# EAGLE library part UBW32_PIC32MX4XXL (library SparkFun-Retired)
Generic PIC32MX4XXL SparkFun Products None
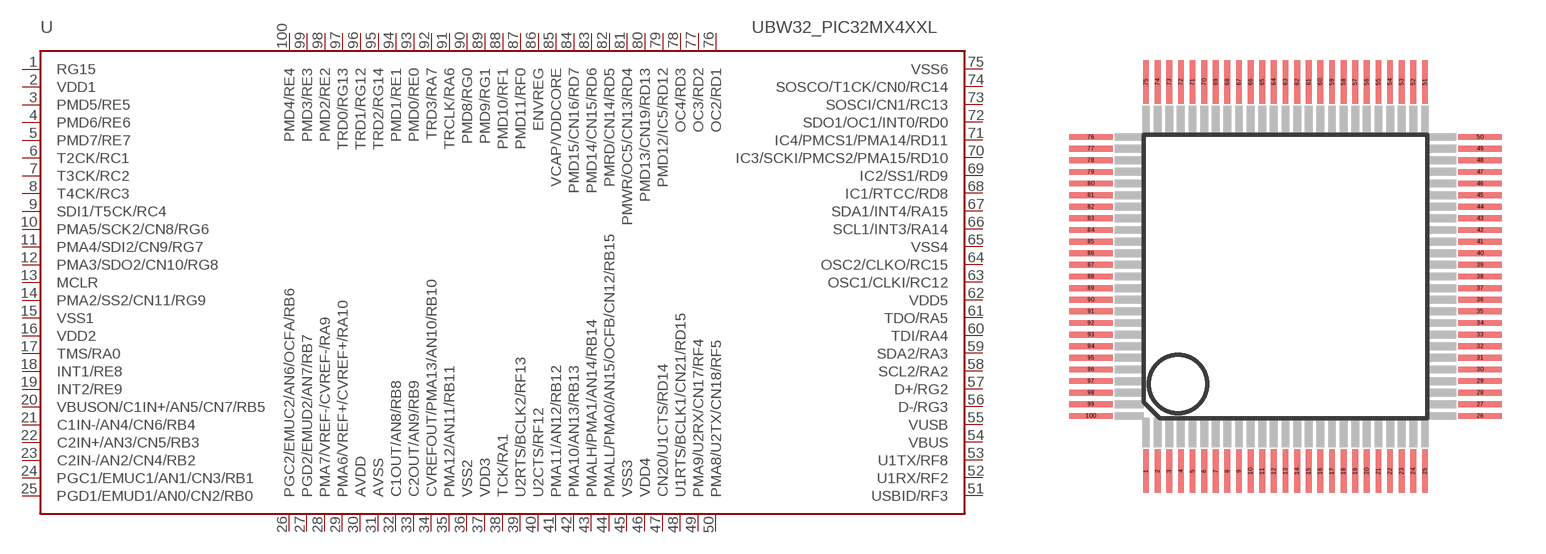
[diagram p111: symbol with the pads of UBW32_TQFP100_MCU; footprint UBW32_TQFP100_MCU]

Designator prefix -

## UBW32_PIC32MX4XXLTQFP100  [UBW32_TQFP100_MCU]
1  RG15
2  VDD1
3  PMD5/RE5
4  PMD6/RE6
5  PMD7/RE7
6  T2CK/RC1
7  T3CK/RC2
8  T4CK/RC3
9  SDI1/T5CK/RC4
10  PMA5/SCK2/CN8/RG6
11  PMA4/SDI2/CN9/RG7
12  PMA3/SDO2/CN10/RG8
13  MCLR
14  PMA2/SS2/CN11/RG9
15  VSS1
16  VDD2
17  TMS/RA0
18  INT1/RE8
19  INT2/RE9
20  VBUSON/C1IN+/AN5/CN7/RB5
21  C1IN-/AN4/CN6/RB4
22  C2IN+/AN3/CN5/RB3
23  C2IN-/AN2/CN4/RB2
24  PGC1/EMUC1/AN1/CN3/RB1
25  PGD1/EMUD1/AN0/CN2/RB0
26  PGC2/EMUC2/AN6/OCFA/RB6
27  PGD2/EMUD2/AN7/RB7
28  PMA7/VREF-/CVREF-/RA9
29  PMA6/VREF+/CVREF+/RA10
30  AVDD
31  AVSS
32  C1OUT/AN8/RB8
33  C2OUT/AN9/RB9
34  CVREFOUT/PMA13/AN10/RB10
35  PMA12/AN11/RB11
36  VSS2
37  VDD3
38  TCK/RA1
39  U2RTS/BCLK2/RF13
40  U2CTS/RF12
41  PMA11/AN12/RB12
42  PMA10/AN13/RB13
43  PMALH/PMA1/AN14/RB14
44  PMALL/PMA0/AN15/OCFB/CN12/RB15
45  VSS3
46  VDD4
47  CN20/U1CTS/RD14
48  U1RTS/BCLK1/CN21/RD15
49  PMA9/U2RX/CN17/RF4
50  PMA8/U2TX/CN18/RF5
51  USBID/RF3
52  U1RX/RF2
53  U1TX/RF8
54  VBUS
55  VUSB
56  D-/RG3
57  D+/RG2
58  SCL2/RA2
59  SDA2/RA3
60  TDI/RA4
61  TDO/RA5
62  VDD5
63  OSC1/CLKI/RC12
64  OSC2/CLKO/RC15
65  VSS4
66  SCL1/INT3/RA14
67  SDA1/INT4/RA15
68  IC1/RTCC/RD8
69  IC2/SS1/RD9
70  IC3/SCKI/PMCS2/PMA15/RD10
71  IC4/PMCS1/PMA14/RD11
72  SDO1/OC1/INT0/RD0
73  SOSCI/CN1/RC13
74  SOSCO/T1CK/CN0/RC14
75  VSS6
76  OC2/RD1
77  OC3/RD2
78  OC4/RD3
79  PMD12/IC5/RD12
80  PMD13/CN19/RD13
81  PMWR/OC5/CN13/RD4
82  PMRD/CN14/RD5
83  PMD14/CN15/RD6
84  PMD15/CN16/RD7
85  VCAP/VDDCORE
86  ENVREG
87  PMD11/RF0
88  PMD10/RF1
89  PMD9/RG1
90  PMD8/RG0
91  TRCLK/RA6
92  TRD3/RA7
93  PMD0/RE0
94  PMD1/RE1
95  TRD2/RG14
96  TRD1/RG12
97  TRD0/RG13
98  PMD2/RE2
99  PMD3/RE3
100  PMD4/RE4

## Footprint UBW32_TQFP100_MCU (pad centres in mm)
Thin Quad Flat Pack
smd 0.2 x 1.5: 1 -4.8,-6.7; 2 -4.4,-6.7; 3 -4,-6.7; 4 -3.6,-6.7; 5 -3.2,-6.7; 6 -2.8,-6.7; 7 -2.4,-6.7; 8 -2,-6.7; 9 -1.6,-6.7; 10 -1.2,-6.7; 11 -0.8,-6.7; 12 -0.4,-6.7; 13 0,-6.7; 14 0.4,-6.7; 15 0.8,-6.7; 16 1.2,-6.7; 17 1.6,-6.7; 18 2,-6.7; 19 2.4,-6.7; 20 2.8,-6.7; 21 3.2,-6.7; 22 3.6,-6.7; 23 4,-6.7; 24 4.4,-6.7; 25 4.8,-6.7; 51 4.8,6.7; 52 4.4,6.7; 53 4,6.7; 54 3.6,6.7; 55 3.2,6.7; 56 2.8,6.7; 57 2.4,6.7; 58 2,6.7; 59 1.6,6.7; 60 1.2,6.7; 61 0.8,6.7; 62 0.4,6.7; 63 0,6.7; 64 -0.4,6.7; 65 -0.8,6.7; 66 -1.2,6.7; 67 -1.6,6.7; 68 -2,6.7; 69 -2.4,6.7; 70 -2.8,6.7; 71 -3.2,6.7; 72 -3.6,6.7; 73 -4,6.7; 74 -4.4,6.7; 75 -4.8,6.7
smd 1.5 x 0.2: 26 6.7,-4.8; 27 6.7,-4.4; 28 6.7,-4; 29 6.7,-3.6; 30 6.7,-3.2; 31 6.7,-2.8; 32 6.7,-2.4; 33 6.7,-2; 34 6.7,-1.6; 35 6.7,-1.2; 36 6.7,-0.8; 37 6.7,-0.4; 38 6.7,0; 39 6.7,0.4; 40 6.7,0.8; 41 6.7,1.2; 42 6.7,1.6; 43 6.7,2; 44 6.7,2.4; 45 6.7,2.8; 46 6.7,3.2; 47 6.7,3.6; 48 6.7,4; 49 6.7,4.4; 50 6.7,4.8; 76 -6.7,4.8; 77 -6.7,4.4; 78 -6.7,4; 79 -6.7,3.6; 80 -6.7,3.2; 81 -6.7,2.8; 82 -6.7,2.4; 83 -6.7,2; 84 -6.7,1.6; 85 -6.7,1.2; 86 -6.7,0.8; 87 -6.7,0.4; 88 -6.7,0; 89 -6.7,-0.4; 90 -6.7,-0.8; 91 -6.7,-1.2; 92 -6.7,-1.6; 93 -6.7,-2; 94 -6.7,-2.4; 95 -6.7,-2.8; 96 -6.7,-3.2; 97 -6.7,-3.6; 98 -6.7,-4; 99 -6.7,-4.4; 100 -6.7,-4.8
